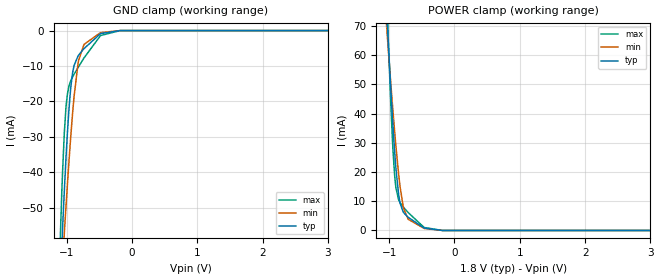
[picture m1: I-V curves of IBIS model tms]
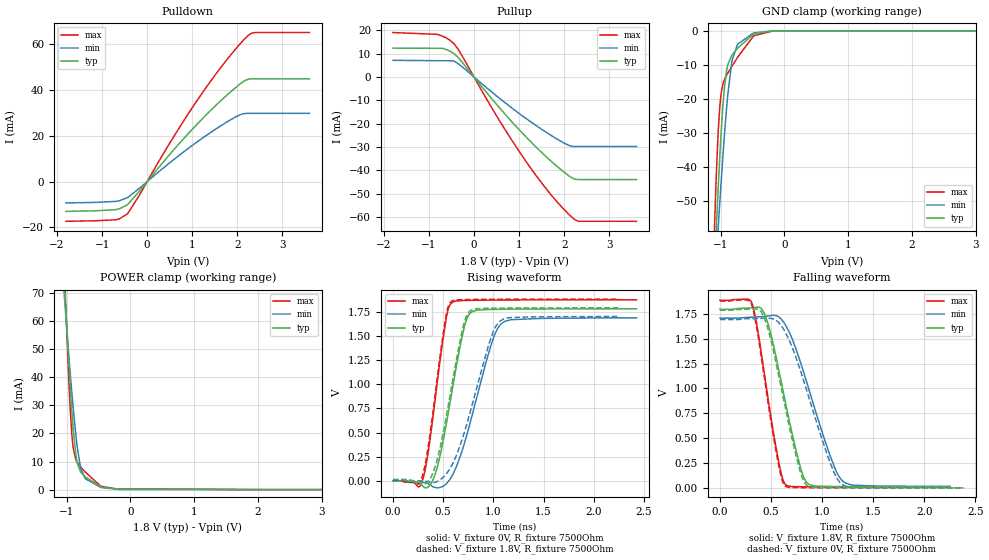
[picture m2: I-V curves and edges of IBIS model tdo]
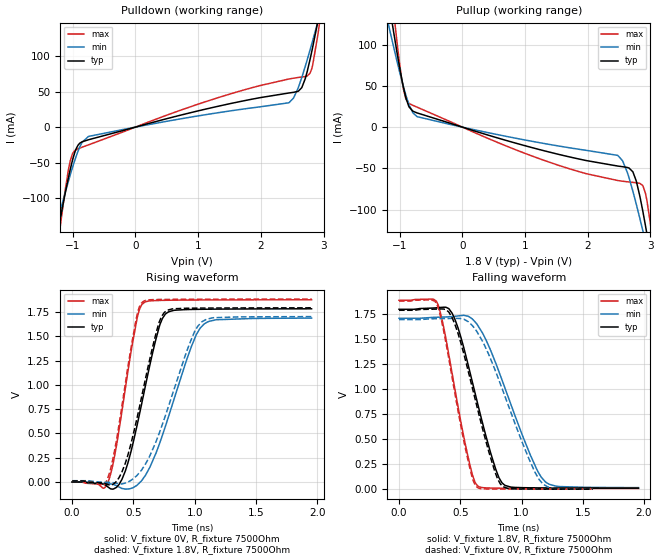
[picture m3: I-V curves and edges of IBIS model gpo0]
|Texas Instruments Incorporated
| DAC38RF8x Dual Channel 14-bit 9 GSPS Digital to Analog Converter
| Marketing part#   Digital Voltage Range   Package-type   #pins
| DAC38RF80/83   1.71V-1.89V   FCBGA   144
[IBIS Ver]   4.1
[File name]   dac38rf80.ibs
[File Rev]   1.0
[Date]   9/6/2016
[Source]
| Texas Instruments Incorporated.
| Analog-eLab Design Center, HPA
| 12500 TI Blvd
| Dallas, TX -75243
[Notes]   Revision History:
| Rev 1.0: 9/6/2016
| - Initial version of the model
| - Model generated from simulations in spectre
| - Model matched to SPICE simulation
| - C_comp although listed in numerical order of value are
|   obtained from varying PVT conditions. For PVT conditions for
|   each specific value refer the buffer description under
|   respective [Model]. IBIS model user is responsible for using
|   appropriate C_comp to simulate for Signal Integrity.
[Disclaimer]
| This model is designed as an aid for customers of Texas Instruments.
| TI and its licensors and suppliers make no warranties, either expressed
| or implied, with respect to this  model, including the warranties of
| merchantability or fitness for a particular purpose. The model is
| provided solely on an "as is" basis. The entire risk as to its quality
| and performance is with the customer.
| For model sync0bn, syncobn_mode5-mode8 have iv-vt mismatch.
|* EXCEPTION:   *
|* - For model gpo0,sdio and tdo Pulldown and Pullup data   *
|*   does not passing through 0 because of (M31.M35,M36) and M12,M13,M14 transistor,R6 resistor   *
|* - For model tdo and sdio there is a leakage in power clamp data   *
|*   because of M1 transistor connected to pad   *
|* - For models sync0bn_mode* Pulldown and pullup data   *
|*   doesnot pass through 0 because of driver switch arrangement   *
|  (M99 M96 M92 M149 M77 M81 M87 M147 M114 M117 M118 M121 M137 M136 M124 M123)-->Pullup   *
|  (M107 M104 M100 M103 M75 M83 M91 M88 M115 M116 M119 M120 M127 M126 M125 M122)->Pulldown   *
[Copyright]
(C) Copyright 2016 Texas Instruments Incorporated.All rights reserved.
|   DAC38RF80
[Component]   DAC38RF80
[Manufacturer]   TI
[Package]   |FCBGA 144
|   typ   min   max
R_pkg   0.01   0.008   0.012
L_pkg   0.1nH   0.08nH   0.12nH
C_pkg   0.1pF   0.08pF   0.12pF
[Pin]  signal_name   model_name   R_pin   L_pin   C_pin
A1   RX7+   nc   na   na   na
A2   DGND   gnd   na   na   na
A3   SYSREF+   nc   na   na   na
A4   SYSREF-   nc   na   na   na
A5   VDDDIG09   power   na   na   na
A6   CLKTX-   nc   na   na   na
A7   CLKTX+   nc   na   na   na
A8   VSSCLK   gnd   na   na   na
A9   DACCLK-   nc   na   na   na
A10   DACCLK+   nc   na   na   na
A11   VSSCLK   gnd   na   na   na
A12   DACCLKSE   nc   na   na   na
B1   RX7-   nc   na   na   na
B2   DGND   gnd   na   na   na
B3   VDDS18   power   na   na   na
B4   VDDS18   power   na   na   na
B5   VDDDIG09   power   na   na   na
B6   VDDTX09   power   na   na   na
B7   VDDTX18   power   na   na   na
B8   VSSCLK   gnd   na   na   na
B9   VDDAPLL18   power   na   na   na
B10   VDDAPLL18   power   na   na   na
B11   VSSCLK   gnd   na   na   na
B12   VSSCLK   gnd   na   na   na
C1   RX6-   nc   na   na   na
C2   DGND   gnd   na   na   na
C3   _SYNC0-   sync0bn   na   na   na
C4   _SYNC0+   sync0bn   na   na   na
C5   VDDDIG09   power   na   na   na
C6   _SYNC1-   sync0bn   na   na   na
C7   _SYNC1+   sync0bn   na   na   na
C8   ATEST   nc   na   na   na
C9   RBIAS   nc   na   na   na
C10   EXTIO   nc   na   na   na
C11   AGND   gnd   na   na   na
C12   AGND   gnd   na   na   na
D1   RX6+   nc   na   na   na
D2   DGND   gnd   na   na   na
D3   IFORCE   nc   na   na   na
D4   VSENSE   nc   na   na   na
D5   VDDDIG09   power   na   na   na
D6   DGND   gnd   na   na   na
D7   VDDDIG09   power   na   na   na
D8   VDDPLL09   power   na   na   na
D9   VDDAVCO18   power   na   na   na
D10   VEE18N   power   na   na   na
D11   AGND   gnd   na   na   na
D12   VOUT2+   nc   na   na   na
E1   RX5+   nc   na   na   na
E2   DGND   gnd   na   na   na
E3   VDDDIG09   power   na   na   na
E4   VDDDIG09   power   na   na   na
E5   VDDDIG09   power   na   na   na
E6   VDDDIG09   power   na   na   na
E7   DGND   gnd   na   na   na
E8   VDDPLL09   power   na   na   na
E9   VDDAVCO18   power   na   na   na
E10   VEE18N   power   na   na   na
E11   AGND   gnd   na   na   na
E12   VOUT2-   nc   na   na   na
F1   RX5-   nc   na   na   na
F2   DGND   gnd   na   na   na
F3   AMUX1   nc   na   na   na
F4   VDDDIG09   power   na   na   na
F5   VDDDIG09   power   na   na   na
F6   DGND   gnd   na   na   na
F7   VDDE09   power   na   na   na
F8   VSSCLK   gnd   na   na   na
F9   VSSCLK   gnd   na   na   na
F10   VSSCLK   gnd   na   na   na
F11   VDDA09   power   na   na   na
F12   AGND   gnd   na   na   na
G1   RX4-   nc   na   na   na
G2   DGND   gnd   na   na   na
G3   AMUX0   nc   na   na   na
G4   VDDDIG09   power   na   na   na
G5   VDDDIG09   power   na   na   na
G6   VDDE09   power   na   na   na
G7   DGND   gnd   na   na   na
G8   VDDL1_09   power   na   na   na
G9   VDDCLK09   power   na   na   na
G10   VDDL2_09   power   na   na   na
G11   VDDA18   power   na   na   na
G12   VDDOUT18   power   na   na   na
H1   RX4+   nc   na   na   na
H2   VDDR18   power   na   na   na
H3   VDDT09   power   na   na   na
H4   TDI   tms   na   na   na
H5   VDDIO18   power   na   na   na
H6   DGND   gnd   na   na   na
H7   VDDE09   power   na   na   na
H8   VDDL1_09   power   na   na   na
H9   VDDCLK09   power   na   na   na
H10   VDDL2_09   power   na   na   na
H11   VDDA18   power   na   na   na
H12   VDDOUT18   nc   na   na   na
J1   RX0+   nc   na   na   na
J2   VDDR18   power   na   na   na
J3   VDDT09   power   na   na   na
J4   TDO   tdo   na   na   na
J5   _TRST   tms   na   na   na
J6   VDDE09   power   na   na   na
J7   DGND   gnd   na   na   na
J8   VSSCLK   gnd   na   na   na
J9   VSSCLK   gnd   na   na   na
J10   VSSCLK   gnd   na   na   na
J11   VDDA09   power   na   na   na
J12   AGND   gnd   na   na   na
K1   RX0-   nc   na   na   na
K2   DGND   gnd   na   na   na
K3   TESTMODE   tms   na   na   na
K4   TCLK   tms   na   na   na
K5   TMS   tms   na   na   na
K6   TXENABLE   tms   na   na   na
K7   GPI0   tms   na   na   na
K8   ALARM   tdo   na   na   na
K9   RESET   tms   na   na   na
K10   VEE18N   power   na   na   na
K11   AGND   gnd   na   na   na
K12   VOUT1-   nc   na   na   na
L1   RX1-   nc   na   na   na
L2   DGND   gnd   na   na   na
L3   DGND   gnd   na   na   na
L4   DGND   gnd   na   na   na
L5   DGND   gnd   na   na   na
L6   GPO1   gpo0   na   na   na
L7   GPO0   gpo0   na   na   na
L8   SLEEP   tms   na   na   na
L9   SCLK   tms   na   na   na
L10   VEE18N   power   na   na   na
L11   AGND   gnd   na   na   na
L12   VOUT1+   nc   na   na   na
M1   RX1+   nc   na   na   na
M2   RX2+   nc   na   na   na
M3   RX2-   nc   na   na   na
M4   RX3-   nc   na   na   na
M5   RX3+   nc   na   na   na
M6   DGND   gnd   na   na   na
M7   GPI1   tms   na   na   na
M8   _SDEN   tms   na   na   na
M9   SDO   tdo   na   na   na
M10   SDIO   sdio   na   na   na
M11   AGND   gnd   na   na   na
M12   AGND   gnd   na   na   na
[Diff_pin]   inv_pin   vdiff   tdelay_typ   tdelay_min   tdelay_max
C4   C3   NA   NA   NA   NA
C7   C6   NA   NA   NA   NA
[Model Selector] sync0bn
sync0bn_mode1   1.8   digital output
sync0bn_mode2   1.8   digital output
sync0bn_mode3   1.8   digital output
sync0bn_mode4   1.8   digital output
| Models and submodels in the file (8): tms (Input), tdo (3-state), gpo0 (Output), sdio (I/O), sync0bn_mode1 (Output), sync0bn_mode2 (Output), sync0bn_mode3 (Output), sync0bn_mode4 (Output)
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|   tms Model
[Model]   tms
Model_type   Input
Vinl = 0.54
Vinh = 1.26
|   typ   min   max
|   (nom PVT)   (fast PVT)   (slow PVT)
C_comp   3.389e-13   3.165e-13   3.551e-13
| Where nom  PVT is Nominal Process, 1.8V, 27C
|   Fast PVT is Strong Process,  1.89V, -40C
|   Slow PVT is Weak Process,   1.71V, 105C
[Model spec]
|subparameter
Vinl   0.54   0.51   0.57
Vinh   1.26   1.19   1.33
[Voltage Range]   1.8   1.71   1.89
|Junction Temperature
[Temperature Range]   27   105   -40
[Power Clamp Reference]   1.8   1.71   1.89
[GND Clamp Reference]   0   0   0
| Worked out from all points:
|   GND clamp passes 1 mA (typ) near -0.49 V on its own axis
|   POWER clamp passes 1 mA (typ) near -0.47 V on its own axis
[GND Clamp]
|   Voltage   I(typ)   I(min)   I(max)
-1.8V     -418.3mA   -319.6mA   -575.1mA
-1.121V   -81.36mA   -84.08mA   -72.77mA
-1.074V   -61.04mA   -69.19mA   -46.05mA
-1.063V   -56.4mA    -65.72mA   -40.54mA
-1.035V   -45.19mA   -57.09mA   -28.82mA
-987.3mV  -28.81mA   -43.4mA    -17.92mA
-934.2mV  -15.73mA   -29.4mA    -14.06mA
-886.9mV  -9.97mA    -18.86mA   -12.36mA
-816.7mV  -6.944mA   -8.464mA   -10.19mA
-732.6mV  -5.062mA   -3.887mA   -7.695mA
-486.4mV  -957.3uA   -644.7uA   -1.557mA
3.6V      0A         0A         0A
[POWER Clamp]
|   Voltage   I(typ)   I(min)   I(max)
-1.8V     456.8mA    335.7mA    653mA
-1.032V   72.92mA    68.13mA    77.91mA
-1.008V   62.44mA    60.63mA    62.8mA
-973.8mV  48.31mA    50.33mA    43.26mA
-938.2mV  34.82mA    40.11mA    26.61mA
-917.4mV  27.77mA    34.45mA    19.56mA
-894.7mV  21.05mA    28.61mA    14.51mA
-842.4mV  10.61mA    16.97mA    9.926mA
-774mV    6.019mA    7.341mA    7.802mA
-707.6mV  4.488mA    3.844mA    6.116mA
-469.4mV  920.9uA    763uA      1.162mA
3.6V      0A         0A         0A
|   tdo Model
[Model]   tdo
Model_type   3-state
Polarity   Non-Inverting
Vmeas = 0.9
Vref = 0
Cref = 2pF
Rref = 100
|   typ   min   max
|   (nom PVT)   (fast PVT)   (slow PVT)
C_comp   2.344e-13   2.236e-13   2.486e-13
| Where nom  PVT is Nominal Process, 1.8V, 27C
|   Fast PVT is Strong Process,  1.89V, -40C
|   Slow PVT is Weak Process,   1.71V, 105C
[Voltage Range]   1.8   1.71   1.89
|Junction Temperature
[Temperature Range]   27   105   -40
[Pullup Reference]   1.8   1.71   1.89
[Pulldown Reference]   0   0   0
[Power Clamp Reference]   1.8   1.71   1.89
[GND Clamp Reference]   0   0   0
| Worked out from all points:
|   slope of the pulldown table from 0 to 0.27 V, typ, clamps not added: 41.5 ohm
|   slope of the pullup table from 0 to 0.27 V, typ, clamps not added: 41.8 ohm
|   GND clamp passes 1 mA (typ) near -0.49 V on its own axis
|   POWER clamp passes 1 mA (typ) near -0.47 V on its own axis
|   falling waveform, V_fixture 1.8V, R_fixture 7500Ohm: 20-80 % time 224ps typ, 314ps min, 171ps max; typ from 1.8 V to 0.011 V
|   rising waveform, V_fixture 0V, R_fixture 7500Ohm: 20-80 % time 186ps typ, 264ps min, 142ps max; typ from 0 V to 1.79 V
|   rising waveform, V_fixture 1.8V, R_fixture 7500Ohm: 20-80 % time 192ps typ, 278ps min, 144ps max; typ from 0.01 V to 1.79 V
|   falling waveform, V_fixture 0V, R_fixture 7500Ohm: 20-80 % time 225ps typ, 320ps min, 171ps max; typ from 1.79 V to 0.001 V
[Pulldown]
|   Voltage   I(typ)   I(min)   I(max)
-1.8V     -12.98mA   -9.299mA   -17.31mA
-700.5mV  -12.23mA   -8.616mA   -16.66mA
-437.4mV  -10.01mA   -6.958mA   -13.99mA
-180mV    -4.338mA   -3.01mA    -6.13mA
554.9mV   13.14mA    9.096mA    18.59mA
1.114V    25.25mA    17.45mA    35.66mA
1.545V    33.75mA    23.29mA    47.61mA
1.976V    41.34mA    28.45mA    58.29mA
2.131V    43.71mA    29.66mA    61.73mA
2.277V    44.88mA    29.85mA    64.41mA
2.392V    44.94mA    29.85mA    65.14mA
3.6V      44.94mA    29.85mA    65.14mA
[GND Clamp]
|   Voltage   I(typ)   I(min)   I(max)
-1.8V     -418.3mA   -319.6mA   -575.1mA
-1.121V   -81.4mA    -84.1mA    -72.83mA
-1.074V   -61.09mA   -69.22mA   -46.11mA
-1.063V   -56.45mA   -65.74mA   -40.6mA
-1.035V   -45.24mA   -57.12mA   -28.89mA
-987.3mV  -28.86mA   -43.43mA   -17.99mA
-934.2mV  -15.78mA   -29.43mA   -14.13mA
-886.9mV  -10.02mA   -18.89mA   -12.43mA
-816.7mV  -6.995mA   -8.499mA   -10.26mA
-732.6mV  -5.114mA   -3.923mA   -7.764mA
-488.3mV  -1.028mA   -692.5uA   -1.66mA
3.6V      0A         0A         0A
[Pullup]
|   Voltage   I(typ)   I(min)   I(max)
-1.8V     12.39mA    7.162mA    19.07mA
-818.5mV  12.32mA    7.009mA    18.32mA
-698.4mV  12.3mA     6.99mA     17.49mA
-461.1mV  10.2mA     6.953mA    14.55mA
-342.8mV  8.128mA    5.586mA    11.55mA
564.4mV   -13.25mA   -9.156mA   -18.78mA
1.112V    -24.93mA   -17.25mA   -35.15mA
1.751V    -36.87mA   -25.58mA   -51.58mA
2.101V    -42.39mA   -29.31mA   -58.9mA
2.218V    -43.68mA   -29.79mA   -60.92mA
2.326V    -43.96mA   -29.81mA   -61.86mA
3.6V      -43.96mA   -29.81mA   -61.86mA
[POWER Clamp]
|   Voltage   I(typ)   I(min)   I(max)
-1.8V     456.8mA    335.7mA    653mA
-1.032V   72.98mA    68.15mA    78.03mA
-1.008V   62.5mA     60.65mA    62.92mA
-973.8mV  48.38mA    50.36mA    43.39mA
-938.2mV  34.89mA    40.14mA    26.74mA
-917.4mV  27.86mA    34.48mA    19.69mA
-894.7mV  21.14mA    28.65mA    14.64mA
-842.4mV  10.7mA     17.01mA    10.06mA
-774mV    6.111mA    7.393mA    7.94mA
-707.6mV  4.583mA    3.902mA    6.257mA
-469.4mV  1.026mA    830.1uA    1.318mA
3.6V      0A         0A         0A
[Ramp]
R_load = 7500
|   typ   min   max
dV/dt_r   1.07154/1.86394e-10   1.01554/2.64382e-10   1.12695/1.41572e-10
dV/dt_f   1.0716/2.2423e-10   1.01565/3.14298e-10   1.12698/1.71075e-10
[Falling Waveform]
V_fixture = 1.8V
V_fixture_min = 1.71V
V_fixture_max = 1.89V
R_fixture = 7500Ohm
|   Time   V(typ)   V(min)   V(max)
0s        1.796V     1.706V     1.885V
318.7ps   1.811V     1.716V     1.841V
455ps     1.7V       1.725V     1.008V
574.5ps   1.19V      1.719V     266.1mV
640.3ps   862.7mV    1.639V     35.37mV
752.6ps   344mV      1.372V     12.13mV
840.4ps   64.56mV    1.091V     10.54mV
1.072ns   14.51mV    342.2mV    9.155mV
1.195ns   13.11mV    74.12mV    8.832mV
2.253ns   10.53mV    15.26mV    7.57mV
[Rising Waveform]
V_fixture = 0V
V_fixture_min = 0V
V_fixture_max = 0V
R_fixture = 7500Ohm
|   Time   V(typ)   V(min)   V(max)
0s        87.83nV    326.2nV    91.32nV
290.1ps   -49.13mV   -17.6mV    -10.78mV
338.4ps   -71.34mV   -25.63mV   214.5mV
434ps     112.8mV    -72.78mV   961.2mV
533.3ps   602.2mV    -29.03mV   1.704V
589.2ps   936.9mV    52.52mV    1.851V
759.4ps   1.728V     567mV      1.872V
970.5ps   1.778V     1.387V     1.875V
1.078ns   1.78V      1.629V     1.876V
2.426ns   1.786V     1.691V     1.878V
[Rising Waveform]
V_fixture = 1.8V
V_fixture_min = 1.71V
V_fixture_max = 1.89V
R_fixture = 7500Ohm
|   Time   V(typ)   V(min)   V(max)
0s        9.681mV    13.25mV    7.188mV
290.1ps   -25.95mV   -2.876mV   37.48mV
347.6ps   -11.36mV   -9.124mV   332.2mV
434ps     193.3mV    -11.1mV    1.013V
529.6ps   658.3mV    67.77mV    1.721V
584.6ps   981.1mV    157.8mV    1.864V
750.8ps   1.744V     645.5mV    1.881V
960.7ps   1.791V     1.433V     1.883V
1.061ns   1.792V     1.652V     1.884V
2.253ns   1.795V     1.705V     1.885V
[Falling Waveform]
V_fixture = 0V
V_fixture_min = 0V
V_fixture_max = 0V
R_fixture = 7500Ohm
|   Time   V(typ)   V(min)   V(max)
0s        1.786V     1.693V     1.878V
304.8ps   1.798V     1.702V     1.858V
359.5ps   1.799V     1.703V     1.611V
455ps     1.65V      1.705V     965.2mV
582.5ps   1.092V     1.652V     188.9mV
640.3ps   805.4mV    1.564V     17.24mV
829.2ps   50.25mV    1.045V     1.943mV
1.061ns   2.136mV    301.5mV    1.433mV
1.177ns   1.756mV    50.36mV    1.297mV
2.384ns   599.6uV    989.6uV    286uV
|   gpo0 Model
[Model]   gpo0
Model_type   Output
Polarity   Non-Inverting
Vmeas = 0.9
Vref = 0
Cref = 2pF
Rref = 100
|   typ   min   max
|   (nom PVT)   (fast PVT)   (slow PVT)
C_comp   2.344e-13   2.236e-13   2.486e-13
| Where nom  PVT is Nominal Process, 1.8V, 27C
|   Fast PVT is Strong Process,  1.89V, -40C
|   Slow PVT is Weak Process,   1.71V, 105C
[Voltage Range]   1.8   1.71   1.89
|Junction Temperature
[Temperature Range]   27   105   -40
[Pullup Reference]   1.8   1.71   1.89
[Pulldown Reference]   0   0   0
[Power Clamp Reference]   1.8   1.71   1.89
[GND Clamp Reference]   0   0   0
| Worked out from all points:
|   slope of the pulldown table from 0 to 0.27 V, typ, clamps not added: 41.3 ohm
|   slope of the pullup table from 0 to 0.27 V, typ, clamps not added: 41.8 ohm
|   falling waveform, V_fixture 1.8V, R_fixture 7500Ohm: 20-80 % time 224ps typ, 314ps min, 171ps max; typ from 1.8 V to 0.011 V
|   rising waveform, V_fixture 0V, R_fixture 7500Ohm: 20-80 % time 186ps typ, 264ps min, 142ps max; typ from 0 V to 1.78 V
|   rising waveform, V_fixture 1.8V, R_fixture 7500Ohm: 20-80 % time 192ps typ, 278ps min, 144ps max; typ from 0.01 V to 1.79 V
|   falling waveform, V_fixture 0V, R_fixture 7500Ohm: 20-80 % time 225ps typ, 319ps min, 171ps max; typ from 1.79 V to 0.001 V
[Pulldown]
|   Voltage   I(typ)   I(min)   I(max)
-1.8V     -429.7mA   -327.5mA   -590.4mA
-1.256V   -156.5mA   -137.4mA   -180.5mA
-1.216V   -137.6mA   -124.1mA   -152.5mA
-1.005V   -47.26mA   -57.45mA   -37.95mA
-914.4mV  -25.44mA   -33.75mA   -30.47mA
-748.3mV  -17.82mA   -13.14mA   -25.05mA
2.448V    48.24mA    34.42mA    67.98mA
2.653V    55.83mA    70.24mA    70.82mA
2.785V    95.8mA     109.2mA    76.19mA
2.91V     149.5mA    149mA      130.8mA
2.977V    180.5mA    171.1mA    174mA
3.6V      482.9mA    382.3mA    624.8mA
[Pullup]
|   Voltage   I(typ)   I(min)   I(max)
-1.8V     469.2mA    342.9mA    672.1mA
-1.148V   140.4mA    114.9mA    177.3mA
-1.033V   86.76mA    77.35mA    97.61mA
-900.4mV  35.91mA    38.99mA    34.41mA
-719.3mV  17.23mA    12.7mA     24.2mA
1.114V    -24.89mA   -17.23mA   -35.09mA
2.478V    -47.24mA   -34.28mA   -64.78mA
2.72V     -54.22mA   -77.7mA    -67.08mA
2.875V    -100.5mA   -124.4mA   -70.69mA
2.921V    -119.9mA   -139.3mA   -80.47mA
3.026V    -166.3mA   -173.2mA   -132.8mA
3.6V      -442.7mA   -367.2mA   -539.6mA
[Ramp]
R_load = 7500
|   typ   min   max
dV/dt_r   1.07154/1.86394e-10   1.01554/2.64382e-10   1.12695/1.41572e-10
dV/dt_f   1.0716/2.2423e-10   1.01565/3.14298e-10   1.12698/1.71075e-10
[Falling Waveform]
V_fixture = 1.8V
V_fixture_min = 1.71V
V_fixture_max = 1.89V
R_fixture = 7500Ohm
|   Time   V(typ)   V(min)   V(max)
0s        1.796V     1.706V     1.885V
318.7ps   1.811V     1.716V     1.841V
455ps     1.7V       1.725V     1.008V
574.5ps   1.19V      1.719V     266.1mV
640.3ps   862.7mV    1.639V     35.37mV
752.6ps   344mV      1.372V     12.13mV
840.4ps   64.56mV    1.091V     10.54mV
1.072ns   14.51mV    342.2mV    9.155mV
1.195ns   13.11mV    74.12mV    8.832mV
1.954ns   10.86mV    16.1mV     7.797mV
[Rising Waveform]
V_fixture = 0V
V_fixture_min = 0V
V_fixture_max = 0V
R_fixture = 7500Ohm
|   Time   V(typ)   V(min)   V(max)
0s        87.83nV    326.2nV    91.32nV
290.1ps   -49.13mV   -17.6mV    -10.78mV
338.4ps   -71.34mV   -25.63mV   214.5mV
434ps     112.8mV    -72.78mV   961.2mV
533.3ps   602.2mV    -29.03mV   1.704V
589.2ps   936.9mV    52.52mV    1.851V
759.4ps   1.728V     567mV      1.872V
970.5ps   1.778V     1.387V     1.875V
1.077ns   1.78V      1.628V     1.876V
1.954ns   1.785V     1.689V     1.878V
[Rising Waveform]
V_fixture = 1.8V
V_fixture_min = 1.71V
V_fixture_max = 1.89V
R_fixture = 7500Ohm
|   Time   V(typ)   V(min)   V(max)
0s        9.681mV    13.25mV    7.188mV
290.1ps   -25.95mV   -2.876mV   37.48mV
347.6ps   -11.36mV   -9.124mV   332.2mV
434ps     193.3mV    -11.1mV    1.013V
529.6ps   658.3mV    67.77mV    1.721V
584.6ps   981.1mV    157.8mV    1.864V
750.8ps   1.744V     645.5mV    1.881V
960.7ps   1.791V     1.433V     1.883V
1.057ns   1.792V     1.649V     1.884V
1.954ns   1.795V     1.704V     1.885V
[Falling Waveform]
V_fixture = 0V
V_fixture_min = 0V
V_fixture_max = 0V
R_fixture = 7500Ohm
|   Time   V(typ)   V(min)   V(max)
0s        1.786V     1.693V     1.878V
304.8ps   1.798V     1.702V     1.858V
359.5ps   1.799V     1.703V     1.611V
455ps     1.65V      1.705V     965.2mV
566.3ps   1.172V     1.671V     271.6mV
634.7ps   833.2mV    1.576V     23.57mV
737.2ps   356.8mV    1.331V     2.586mV
829.2ps   50.25mV    1.045V     1.943mV
1.143ns   1.843mV    97.28mV    1.334mV
1.581ns   1.203mV    1.845mV    890.7uV
